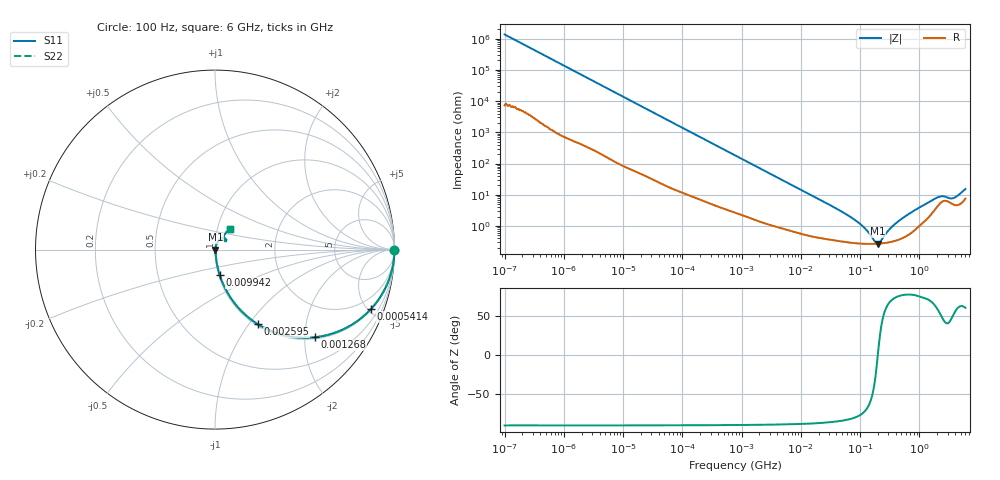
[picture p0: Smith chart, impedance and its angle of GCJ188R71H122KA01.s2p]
!Murata Part Number: GCJ188R71H122KA01
!These Parameters are Measured in Series Mode Connection
!Data Generated on Mar 13, 2026
!  o--ll--o
!Port1  Port2
!  o------o
!Operation Temp=25[degC], DC Bias Voltage=0[V]
!Freq. Start=100[Hz] Stop=6[GHz] 401[Steps]
# Hz S RI R 50
!Freq.(Hz) S11(Real) S11(Imag) S21(Real) S21(Imag) S12(Real) S12(Imag) S22(Real) S22(Imag)
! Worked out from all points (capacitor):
!   401 points, 100 Hz to 6 GHz, reference 50 ohm
!   read as one part in series: C = 1.17 nF near 109 Hz
!   lowest |Z| = 271 mohm at 199.7 MHz (marker M1)
!   series resonance near 199.2 MHz, so ESL is about 550 pH
!   S11 on the Smith chart (normalised r, x): 100 Hz: open; 541.4 kHz: 1.07, -5.23; 1.268 MHz: 1.04, -2.25; 2.595 MHz: 1.02, -1.11; 9.942 MHz: 1.01, -0.29; 6 GHz: 1.15, +0.27
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100  1 -7.34e-05  4e-07 7.34e-05  4e-07 7.34e-05  1 -7.34e-05
150  1 -0.00011  8e-07 0.00011  8e-07 0.00011  1 -0.00011
2008  1 -0.00146  1.07e-05 0.00146  1.07e-05 0.00146  1 -0.00146
40335  0.999 -0.0289  0.00104 0.0289  0.00104 0.0289  0.999 -0.0289
169018  0.9846 -0.1184  0.0154 0.1184  0.0154 0.1184  0.9846 -0.1184
541393  0.869 -0.3309  0.131 0.3309  0.131 0.3309  0.869 -0.3309
774597  0.7671 -0.4154  0.2329 0.4154  0.2329 0.4154  0.7671 -0.4154
1267578  0.5574 -0.4883  0.4426 0.4883  0.4426 0.4883  0.5574 -0.4883
2594782  0.2389 -0.4159  0.7611 0.4159  0.7611 0.4159  0.2389 -0.4159
4643984  0.0945 -0.2791  0.9055 0.2791  0.9055 0.2791  0.0945 -0.2791
9941735  0.0263 -0.1418  0.9737 0.1418  0.9737 0.1418  0.0263 -0.1418
1.555665e7  0.0132 -0.0922  0.9868 0.0922  0.9868 0.0922  0.0132 -0.0922
8.154455e7  0.00305 -0.0154  0.9969 0.0154  0.9969 0.0154  0.00305 -0.0154
1.166697e8  0.00276 -0.00852  0.9972 0.00852  0.9972 0.00852  0.00276 -0.00852
1.745687e8  0.00268 -0.00202  0.9973 0.00202  0.9973 0.00202  0.00268 -0.00202
1.996653e8  0.0027 3.88e-05  0.9973 -3.88e-05  0.9973 -3.88e-05  0.0027 3.88e-05
3.124326e8  0.00305 0.00713  0.9969 -0.00713  0.9969 -0.00713  0.00305 0.00713
5.847788e8  0.00494 0.02  0.9951 -0.02  0.9951 -0.02  0.00494 0.02
1.791126e9  0.0344 0.0619  0.9656 -0.0619  0.9656 -0.0619  0.0344 0.0619
2.34314e9  0.058 0.0612  0.942 -0.0612  0.942 -0.0612  0.058 0.0612
3.666503e9  0.0503 0.0533  0.9497 -0.0533  0.9497 -0.0533  0.0503 0.0533
6e9  0.0842 0.1135  0.9158 -0.1135  0.9158 -0.1135  0.0842 0.1135
